(* Logix 5000 AddOnInstructionDefinition export T2CON; software revision 32.02 *)

TYPE Exlar_Control :   // Tritex II Control
STRUCT
   EnableOutputs : INT;   // EnableOutputs
   InputEventsMode : INT;   // 4316
   InputEventsModeLevel : INT;   // 4318
   InputEventsMotion : INT;   // 4317
   HostCommandControlMode : INT;   // 4303
   HostPosition_low : INT;   // 4304
   HostPosition_high : INT;
   HostVelocity_low : INT;   // 4306
   HostVelocity_high : INT;
   HostAcceleration_low : INT;   // 4308
   HostAcceleration_high : INT;
   HostCurrent : INT;   // 4310
   InputEventsMoveEdge : INT;   // 4319
   JogSlowVelocity_low : INT;   // 6022
   JogSlowVelocity_high : INT;
   JogAcceleration_low : INT;   // 6026
   JogAcceleration_high : INT;
   MoveOption : INT;   // 6100
   MoveCurrentLimit : INT;   // 6101
   MoveAcceleration_low : INT;   // 6102
   MoveAcceleration_high : INT;
   MoveDeceleration_low : INT;   // 6500
   MoveDeceleration_high : INT;
   MovePrimaryOption : INT;   // 6106
   spare : INT;   // spare
   MovePrimaryPosition_low : INT;   // 6108
   MovePrimaryPosition_high : INT;
   MovePrimaryVelocity_low : INT;   // 6110
   MovePrimaryVelocity_high : INT;
   MoveSecondaryOption : INT;   // 6112
   spare2 : INT;   // spare
   MoveSecondaryPosition_low : INT;   // 6114
   MoveSecondaryPosition_high : INT;
   MoveSecondaryVelocity_low : INT;   // 6116
   MoveSecondaryVelocity_high : INT;
END_STRUCT
END_TYPE

TYPE Exlar_Drive :   // Tritex II Data
STRUCT
   Control : Exlar_Control;   // Control bits to send to the drive
   Status : Exlar_Status;   // Status bits received from the drive
END_STRUCT
END_TYPE

TYPE Exlar_Status :   // Tritex II Status
STRUCT
   EIP_Comm : INT;   // EIP module communication
   OutputEventsStatus : INT;   // 104
   OutputEventsMoveInPosition : INT;   // 108
   OutputEventsMotion : INT;   // 105
   OutputsEventsMotionActive : INT;   // 107
   PositionFeedback_low : INT;   // 378
   PositionFeedback_high : INT;
   SoftFaults : INT;   // 7
   HardFaults : INT;   // 6
   VelocityDisplay_low : INT;   // 356
   VelocityDisplay_high : INT;
   CurrentDisplay : INT;   // 567
   CurrentContinuous : INT;   // 565
   CurrentLimit : INT;   // 5108
   VoltageHallBattery : INT;   // 8
   VoltageBus : INT;   // 571
   TemperatureBoard : INT;   // 11
   TemperatureActuator : INT;   // 15
END_STRUCT
END_TYPE

ADD_ON_INSTRUCTION T2CON   (* revision 1.0, vendor Exlar Corporation *)
// Help:
// Use the Tritex 2 Control (T2CON) instruction to send commands to drive.
// Module commands includes enabling the drive, defining Home and Motion commands like Stop and Pause.
// Configured for Exlar EIP AOI. 07/01/2014
// ----------------------------------------------------------------------------------------------------------------------------
// Parameters Bit Definition
// ----------------------------------------------------------------------------------------------------------------------------
// Module:  (Input) Tritex 2 Module Commands
// ------------------------------------------------------------------
//      Module.0:     Enable Momentary
//      Module.1:     Enable Maintained
//      Module.2:     Define Home
//      Module.3:     Brake Override
//      Module.4:     Fault Reset
// Motion:  (Input) Tritex 2 Motion Commands
// ------------------------------------------------------------------
//      Motion.0:     Stop Motion
//      Motion.1:     Pause Move
//      Motion.2:     Initiate Home Move
//      Motion.3:     Emergency Move
VAR_IN_OUT
   Drive : Exlar_Drive; {required}   // Drive
END_VAR
VAR_INPUT
   Module : INT; {visible}   // Module Commands
        .0   // Enable Momentary
        .1   // Enable Maintained
        .2   // Define Home
        .3   // Brake Override
        .4   // Fault Reset
   Motion : INT; {visible}   // Motion Commands
        .0   // Stop Motion
        .1   // Pause Move
        .2   // Initiate Home Move
        .3   // Emergency Move
END_VAR
VAR_OUTPUT
   DF : BOOL; {access Read Only, visible}   // Indicates one or more Drive Faults are Active
END_VAR

ROUTINE Logic   (* structured text *)
   (***********************************************)
   (*   Exlar Tritex 2 Control                    *)
   (*                                             *)
   (***********************************************)
   
   (********** Inputs ***********)
   
   (* Module Register *)
   	(* 4316.0 Enable Momentary *)
   	if Module.0	then
   		Drive.Control.InputEventsMode.0	:= 1;
   	else
   		Drive.Control.InputEventsMode.0 := 0;
   	end_if;
   
   	(* 4316.1 Enable Maintained *)
   	if Module.1	then
   		Drive.Control.InputEventsMode.1	:= 1;
   	else
   		Drive.Control.InputEventsMode.1	 := 0;
   	end_if;
   
   	(* 4316.10 Define Home *)
   	if Module.2	then
   		Drive.Control.InputEventsMode.10 := 1;
   	else
   		Drive.Control.InputEventsMode.10 := 0;
   	end_if;
   
   	(* 4316.14 Brake Override *)
   	if Module.3	then
   		Drive.Control.InputEventsMode.14 := 1;
   	else
   		Drive.Control.InputEventsMode.14 := 0;
   	end_if;
   
   	(* 4316.15 Fault Reset *)
   	if Module.4	then
   		Drive.Control.InputEventsMode.15 := 1;
   	else
   		Drive.Control.InputEventsMode.15 := 0;
   	end_if;
   
   (* Motion Register *)
   	(* 4317.2 Stop Motion *)
   	if Motion.0	then
   		Drive.Control.InputEventsMotion.2 := 1;
   	else
   		Drive.Control.InputEventsMotion.2  := 0;
   	end_if;
   
   	(* 4317.3 Pause Move *)
   	if Motion.1	then
   		Drive.Control.InputEventsMotion.3 := 1;
   	else
   		Drive.Control.InputEventsMotion.3 := 0;
   	end_if;
   
   	(* 4317.8 Initiate Home Move *)
   	if Motion.2	then
   		Drive.Control.InputEventsMotion.8:= 1;
   	else
   		Drive.Control.InputEventsMotion.8 := 0;
   	end_if;
   
   	(* 4317.10 Dedicated Position EMove *)
   	if Motion.3	then
   		Drive.Control.InputEventsMotion.10 := 1;
   	else
   		Drive.Control.InputEventsMotion.10  := 0;
   	end_if;
   
   (*********** OUTPUTS  ***********)
   
   (* Drive Faults Active *)
   	If Drive.Control.InputEventsMode.3 then
    		DF := 1;
   	Else
   		DF := 0;
   	End_If;
   
END_ROUTINE
END_ADD_ON_INSTRUCTION
